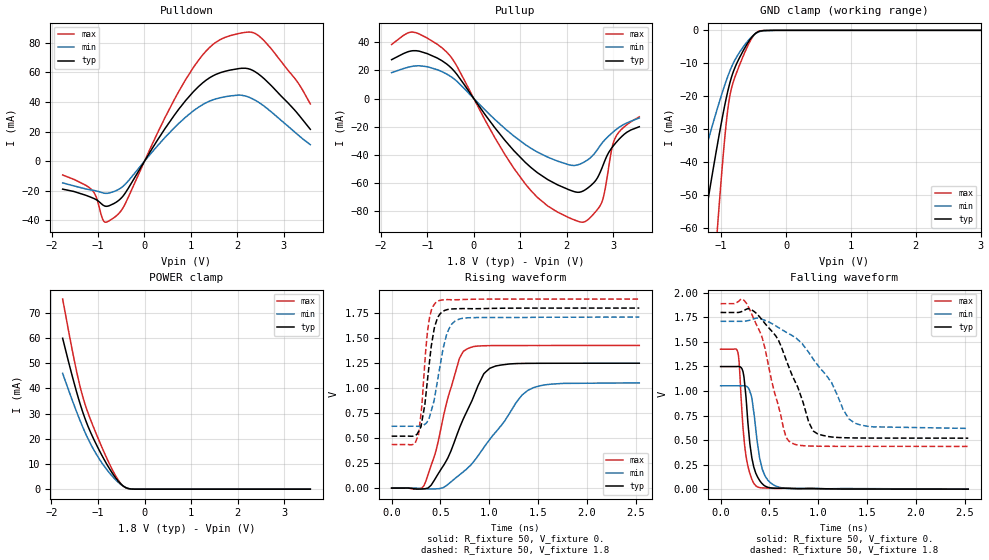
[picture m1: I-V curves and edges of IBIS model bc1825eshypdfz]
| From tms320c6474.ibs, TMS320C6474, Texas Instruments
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|30OHM_5PER_FULLTERM_1P8;
|   MODEL bc1825eshypdfz
[Model] bc1825eshypdfz
Model_type I/O
|C_comp_off 1.025p 974.57f 1.043p
|C_comp_on 899.99f 842.153f 918.882f
C_comp 962.474f 908.362f 980.897f
|Rth_i 16.775Meg NAN 36.892Meg
|Rth_r 23.374 32.235 17.647
|Rth_f 21.657 29.516 16.232
Vinl = 0.630
Vinh = 1.170
Vmeas = 0.9
Cref = 5pF
[Model Spec]
||   Typ   Min   Max
S_overshoot_high   2.100   2.010   2.190
Vinh   1.170   1.111   1.229
Vmeas   0.900   0.855   0.945
Vinl   0.630   0.599   0.662
S_overshoot_low   -0.300  -0.300  -0.300
[Receiver Thresholds]
Vth   = 0.900V
Vth_min = 0.855V
Vth_max = 0.945V
Vinh_ac = +270mV   || Undefined so set to Vinh_dc level
Vinh_dc = +270mV
Vinl_dc = -270mV
Vinl_ac = -270mV   || Undefined so set to Vinl_dc level
Tslew_ac = 5.0ns   || Undefined in specification - set to large value
|| Pointer to HSPICE models:
|ff ti_bc1825eshypdfz.mod ti_bc1825eshypdfz_ff
|tt ti_bc1825eshypdfz.mod ti_bc1825eshypdfz_tt
|ss ti_bc1825eshypdfz.mod ti_bc1825eshypdfz_ss
|| Spice2IBIS controls:
|View_IV No
[Temperature Range]  25   105   -40
|corevdd   1.100  1.045  1.155
[Voltage Range]   1.8   1.71   1.89
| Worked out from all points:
|   slope of the pulldown table from 0 to 0.27 V, typ, clamps not added: 19.6 ohm
|   slope of the pullup table from 0 to 0.27 V, typ, clamps not added: 21.3 ohm
|   GND clamp passes 1 mA (typ) near -0.47 V on its own axis
|   POWER clamp passes 1 mA (typ) near -0.44 V on its own axis
|   rising waveform, R_fixture 50, V_fixture 0.: 20-80 % time 328ps typ, 477ps min, 223ps max; typ from 0 V to 1.25 V
|   rising waveform, R_fixture 50, V_fixture 1.8: 20-80 % time 97.6ps typ, 128ps min, 73.7ps max; typ from 0.519 V to 1.8 V
|   falling waveform, R_fixture 50, V_fixture 0.: 20-80 % time 80.6ps typ, 93.4ps min, 70.5ps max; typ from 1.25 V to 0 V
|   falling waveform, R_fixture 50, V_fixture 1.8: 20-80 % time 300ps typ, 419ps min, 218ps max; typ from 1.8 V to 0.52 V
[Pulldown]
-1.76V    -18.87mA   -14.66mA   -9.325mA
-1.13V    -24.63mA   -19.54mA   -19.47mA
-860.5mV  -30.2mA    -21.62mA   -40.97mA
-607.4mV  -27.67mA   -19.84mA   -36.96mA
-429.6mV  -22.21mA   -16.04mA   -29.67mA
890mV     41.15mA    29.87mA    55.34mA
1.407V    56.46mA    40.66mA    77.01mA
1.843V    61.52mA    44.07mA    84.8mA
2.28V     61.99mA    42.78mA    87.15mA
2.517V    57.24mA    38.48mA    83.07mA
3.276V    32.83mA    18.47mA    54.13mA
3.567V    21.51mA    11.15mA    38.67mA
[Pullup]
-1.767V   27.7mA     18.44mA    38.55mA
-1.309V   34.09mA    23.03mA    47.37mA
-587.4mV  24.73mA    17.54mA    33.28mA
673mV     -29.95mA   -21.52mA   -40.1mA
1.109V    -45.58mA   -32.86mA   -60.92mA
1.594V    -57.88mA   -41.87mA   -76.7mA
2.273V    -66.82mA   -46.9mA    -87.88mA
2.58V     -60.11mA   -39.86mA   -82.27mA
2.752V    -49.96mA   -32.1mA    -74.16mA
2.973V    -35.01mA   -24.6mA    -35.25mA
3.059V    -31.45mA   -22.17mA   -27.03mA
3.56V     -20.12mA   -13.86mA   -13.04mA
[GND Clamp]
-1.76V    -120.2mA   -77.13mA   -249.9mA
-1.521V   -90.24mA   -57.76mA   -187.4mA
-1.322V   -65.76mA   -42.28mA   -132.8mA
-1.234V   -55.07mA   -35.75mA   -108.1mA
-1.057V   -34.51mA   -23.57mA   -59.78mA
-932.9mV  -21.61mA   -15.89mA   -30.24mA
-893.1mV  -18.07mA   -13.71mA   -23.31mA
-853.3mV  -15.04mA   -11.73mA   -18.63mA
-786.9mV  -11.25mA   -8.972mA   -14.13mA
-627.7mV  -5.052mA   -4.189mA   -6.314mA
-437.5mV  -518.7uA   -625.7uA   -437uA
3.567V    0A         0A         0A
[Power Clamp]
-1.76V    59.91mA    45.97mA    75.49mA
-1.582V   46.89mA    36.74mA    57.87mA
-1.467V   39mA       31.02mA    47.3mA
-1.367V   32.81mA    26.37mA    39.4mA
-1.268V   27.44mA    22.09mA    33.07mA
-1.021V   17.16mA    13.42mA    21.2mA
-764.6mV  8.451mA    6.671mA    10.39mA
-597mV    3.878mA    3.261mA    4.513mA
-450.3mV  1.139mA    1.112mA    1.086mA
-350.7mV  261.8uA    304uA      205.5uA
-225mV    10.26uA    20.18uA    5.761uA
3.56V     0A         0A         0A
[Ramp]
dV/dt_r .749/327.937p .632/477.339p .856/223.05p
dV/dt_f .768/300.092p .655/418.977p .873/217.55p
[Rising Waveform]
R_fixture = 50
V_fixture = 0.
0s        0V         1.299uV    0V
330ps     -7.403mV   -6.896mV   23.37mV
455ps     107.9mV    -7.198mV   377.3mV
545ps     247.9mV    15.26mV    780.4mV
695ps     601.2mV    132.6mV    1.299V
770ps     766.5mV    192.5mV    1.39V
940ps     1.136V     400.2mV    1.423V
1.005ns   1.198V     487.3mV    1.424V
1.395ns   1.247V     977.5mV    1.426V
2.535ns   1.249V     1.052V     1.426V
[Rising Waveform]
R_fixture = 50
V_fixture = 1.8
V_fixture_min = 1.71
V_fixture_max = 1.89
0s        519.2mV    618.2mV    435.6mV
275ps     565.6mV    617.9mV    532.9mV
310ps     667.2mV    623.7mV    830.7mV
340ps     833.8mV    638.7mV    1.255V
385ps     1.239V     701.3mV    1.686V
435ps     1.59V      877.3mV    1.834V
475ps     1.711V     1.105V     1.87V
570ps     1.785V     1.556V     1.884V
695ps     1.794V     1.69V      1.884V
2.535ns   1.8V       1.71V      1.89V
[Falling Waveform]
R_fixture = 50
V_fixture = 0.
0s        1.249V     1.053V     1.426V
175ps     1.25V      1.053V     1.399V
190ps     1.25V      1.053V     1.292V
230ps     1.196V     1.054V     617.9mV
265ps     873mV      1.049V     310mV
315ps     354.1mV    949.6mV    114.9mV
375ps     131.6mV    483.9mV    24.59mV
455ps     31.76mV    134mV      11.99mV
610ps     9.773mV    16.85mV    7.19mV
2.535ns   194.1uV    473.5uV    44.24uV
[Falling Waveform]
R_fixture = 50
V_fixture = 1.8
V_fixture_min = 1.71
V_fixture_max = 1.89
0s        1.8V       1.71V      1.89V
210ps     1.807V     1.71V      1.937V
290ps     1.837V     1.719V     1.847V
425ps     1.724V     1.73V      1.546V
570ps     1.553V     1.661V     924.2mV
645ps     1.387V     1.614V     618.8mV
705ps     1.229V     1.58V      485mV
950ps     591mV      1.323V     438.4mV
1.375ns   521.7mV    672.6mV    436.2mV
2.535ns   519.6mV    618.8mV    435.7mV
